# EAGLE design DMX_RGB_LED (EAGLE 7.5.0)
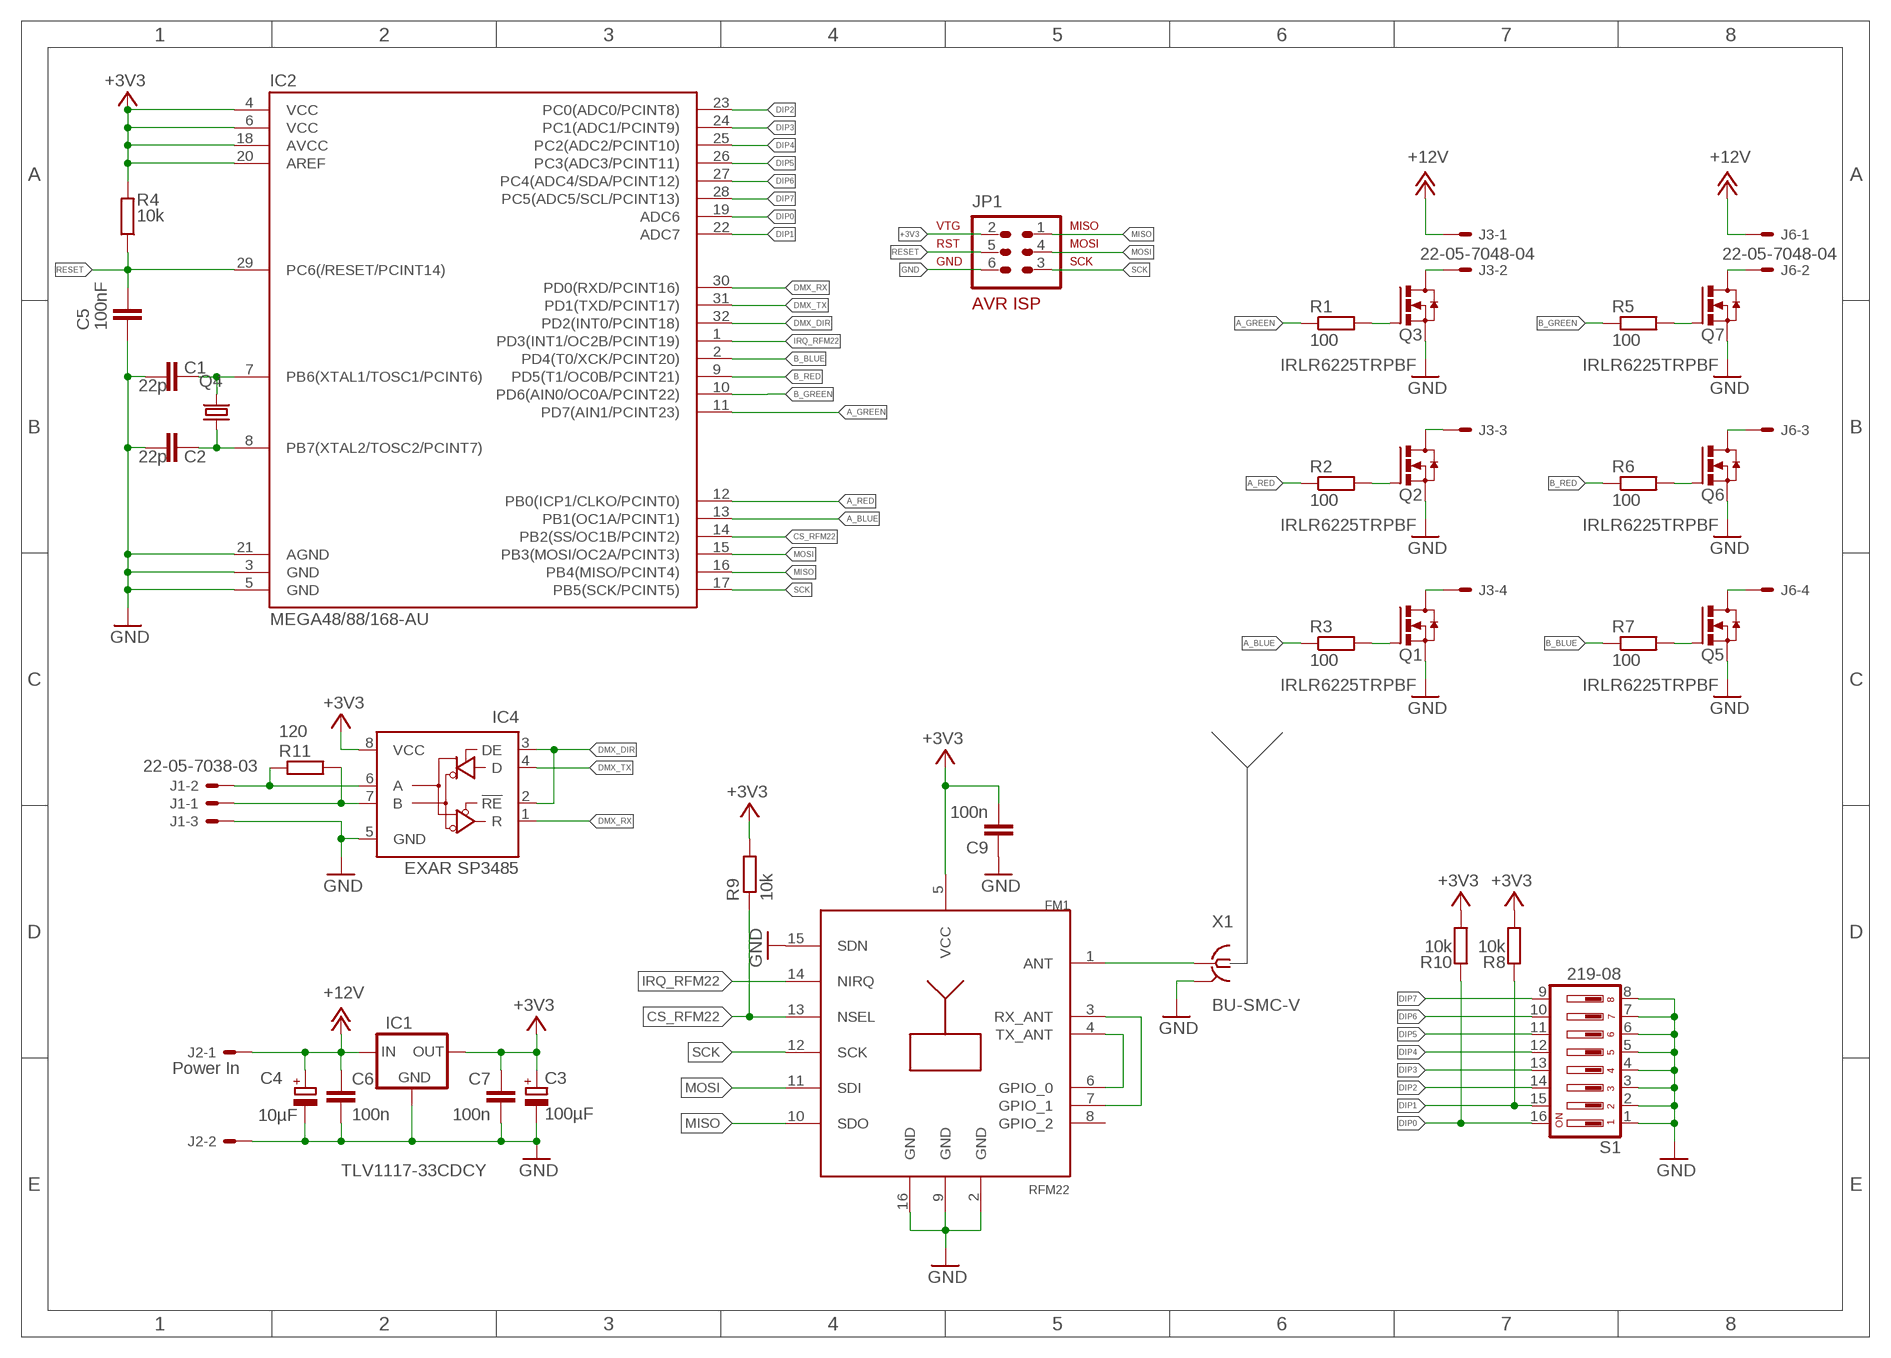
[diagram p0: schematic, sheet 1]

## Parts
C1  22p  C-EUC0805  [C0805]
C2  22p  C-EUC0805  [C0805]
C3  100µF  CPOL-EUSMCD  [SMC_D]
C4  10µF  CPOL-EUSMCD  [SMC_D]
C5  100nF  C-EUC0805  [C0805]
C6  100n  C-EUC0805  [C0805]
C7  100n  C-EUC0805  [C0805]
C9  100n  C-EUC0805  [C0805]
FM1  RFM22  [RFM22]
IC1  TLV1117-33CDCY  [DPACK]
IC2  MEGA48/88/168-AU  [TQFP32-08]
IC4  EXAR SP3485  75176AD  [D_R-PDSO-G8]
J1  22-05-7038-03  [7395-03]
J2  Power In  22-05-7028-02  [7395-02]
J3  22-05-7048-04  [7395-04]
J6  22-05-7048-04  [7395-04]
JP1  AVR-ISP-6  [AVR-ISP-6]
Q1  IRLR6225TRPBF  IRFR1205  [D-PAK_TO252AA]
Q2  IRLR6225TRPBF  IRFR1205  [D-PAK_TO252AA]
Q3  IRLR6225TRPBF  IRFR1205  [D-PAK_TO252AA]
Q4  CRYSTALCTS406  [CTS406]
Q5  IRLR6225TRPBF  IRFR1205  [D-PAK_TO252AA]
Q6  IRLR6225TRPBF  IRFR1205  [D-PAK_TO252AA]
Q7  IRLR6225TRPBF  IRFR1205  [D-PAK_TO252AA]
R1  100  R-EU_R0805  [R0805]
R2  100  R-EU_R0805  [R0805]
R3  100  R-EU_R0805  [R0805]
R4  10k  R-EU_R0805  [R0805]
R5  100  R-EU_R0805  [R0805]
R6  100  R-EU_R0805  [R0805]
R7  100  R-EU_R0805  [R0805]
R8  10k  R-EU_R0805  [R0805]
R9  10k  R-EU_R0805  [R0805]
R10  10k  R-EU_R0805  [R0805]
R11  120  R-EU_R0805  [R0805]
S1  219-08  [CTS-219-08]
X1  BU-SMC-V  [BU-SMC-V]

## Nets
+3V3: C3.+ C7.1 C9.2 FM1.5(VCC) IC1.4(OUT) IC2.4(VCC) IC2.6(VCC) IC2.18(AVCC) IC2.20(AREF) IC4.8(VCC) JP1.2 R4.2 R8.1 R9.2 R10.1
+12V: C4.+ C6.1 IC1.3(IN) J2.1 J3.1 J6.1
A_BLUE: IC2.13(PB1(OC1A/PCINT1)) R3.1
A_GREEN: IC2.11(PD7(AIN1/PCINT23)) R1.1
A_RED: IC2.12(PB0(ICP1/CLKO/PCINT0)) R2.1
B_BLUE: IC2.2(PD4(T0/XCK/PCINT20)) R7.1
B_GREEN: IC2.10(PD6(AIN0/OC0A/PCINT22)) R5.1
B_RED: IC2.9(PD5(T1/OC0B/PCINT21)) R6.1
CS_RFM22: FM1.13(NSEL) IC2.14(PB2(SS/OC1B/PCINT2)) R9.1
DIP0: IC2.19(ADC6) R10.2 S1.16
DIP1: IC2.22(ADC7) R8.2 S1.15
DIP2: IC2.23(PC0(ADC0/PCINT8)) S1.14
DIP3: IC2.24(PC1(ADC1/PCINT9)) S1.13
DIP4: IC2.25(PC2(ADC2/PCINT10)) S1.12
DIP5: IC2.26(PC3(ADC3/PCINT11)) S1.11
DIP6: IC2.27(PC4(ADC4/SDA/PCINT12)) S1.10
DIP7: IC2.28(PC5(ADC5/SCL/PCINT13)) S1.9
DMX_DIR: IC2.32(PD2(INT0/PCINT18)) IC4.2(!RE) IC4.3(DE)
DMX_RX: IC2.30(PD0(RXD/PCINT16)) IC4.1(R)
DMX_TX: IC2.31(PD1(TXD/PCINT17)) IC4.4(D)
GND: C1.1 C2.2 C3.- C4.- C5.1 C6.2 C7.2 C9.1 FM1.2(GND) FM1.9(GND) FM1.15(SDN) FM1.16(GND) IC1.1(GND) IC2.3(GND) IC2.5(GND) IC2.21(AGND) IC4.5(GND) J1.3 J2.2 JP1.6 Q1.3(S) Q2.3(S) Q3.3(S) Q5.3(S) Q6.3(S) Q7.3(S) S1.1 S1.2 S1.3 S1.4 S1.5 S1.6 S1.7 S1.8 X1.2(GND)
IRQ_RFM22: FM1.14(NIRQ) IC2.1(PD3(INT1/OC2B/PCINT19))
MISO: FM1.10(SDO) IC2.16(PB4(MISO/PCINT4)) JP1.1
MOSI: FM1.11(SDI) IC2.15(PB3(MOSI/OC2A/PCINT3)) JP1.4
N$1: Q1.1(G) R3.2
N$2: Q2.1(G) R2.2
N$3: Q3.1(G) R1.2
N$4: Q5.1(G) R7.2
N$5: Q6.1(G) R6.2
N$6: Q7.1(G) R5.2
N$8: J6.2 Q7.4(D)
N$9: J6.3 Q6.4(D)
N$10: J6.4 Q5.4(D)
N$11: FM1.1(ANT) X1.1
N$13: FM1.4(TX_ANT) FM1.6(GPIO_0)
N$14: C2.1 IC2.8(PB7(XTAL2/TOSC2/PCINT7)) Q4.1
N$15: FM1.3(RX_ANT) FM1.7(GPIO_1)
N$16: C1.2 IC2.7(PB6(XTAL1/TOSC1/PCINT6)) Q4.3
N$23: J3.2 Q3.4(D)
N$24: J3.3 Q2.4(D)
N$25: IC4.6(A) J1.2 R11.1
N$26: IC4.7(B) J1.1 R11.2
N$27: J3.4 Q1.4(D)
RESET: C5.2 IC2.29(PC6(/RESET/PCINT14)) JP1.5 R4.1
SCK: FM1.12(SCK) IC2.17(PB5(SCK/PCINT5)) JP1.3
Unconnected: FM1.8(GPIO_2)

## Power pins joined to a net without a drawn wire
GND: X1.3(GND) X1.4(GND) X1.5(GND)

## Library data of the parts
C1 C2 C5-C7 C9 = rcl:C-EU: CAPACITOR, European symbol
C3 C4 = rcl:CPOL-EU: POLARIZED CAPACITOR, European symbol
FM1 = RFMxx:RFM22
IC1 = bauteile:TLV1117-33CDCY: 500 mA Adjustable Output Positive Voltage Regulator Source: http://www.onsemi.co.jp .. LM317M-D.PDF
IC2 = bauteile:MEGA48/88/168
IC4 = 751xx:75176A: DIFFERENTIAL BUS TRANSCEIVER Source: http://focus.ti.com/lit/ds/symlink/sn75176a.pdf
J1 = con-molex:22-?-03: CONNECTOR wire to board 2.54 mm (.1 inch) pitch header; OC_FARNELL: unknown; OC_NEWARK: unknown
J2 = con-molex:22-?-02: CONNECTOR; OC_FARNELL: 9731601; OC_NEWARK: unknown
J3 J6 = con-molex:22-?-04: CONNECTOR wire to board 2.54 mm (.1 inch) pitch header; OC_FARNELL: unknown; OC_NEWARK: unknown
JP1 = avr-4:AVR-ISP-6: AVR ISP-6 Serial Programming Header
Q1-Q3 Q5-Q7 = transistor-power:IRFR1205
Q4 = crystal:CRYSTAL: CRYSTAL; OC_FARNELL: unknown; OC_NEWARK: unknown
R1-R11 = rcl:R-EU_: RESISTOR, European symbol
S1 = switch-dil:219-08*: Surface Mount DIP Switch Series 219 SMT CTS Electronic Components Sourc: www.ctscorp.com; OC_FARNELL: unknown; OC_NEWARK: unknown
X1 = con-coax:BU-SMC-V: FEMALE SMC CONNECTOR Radiall R112 426 distributor RS 295-5429

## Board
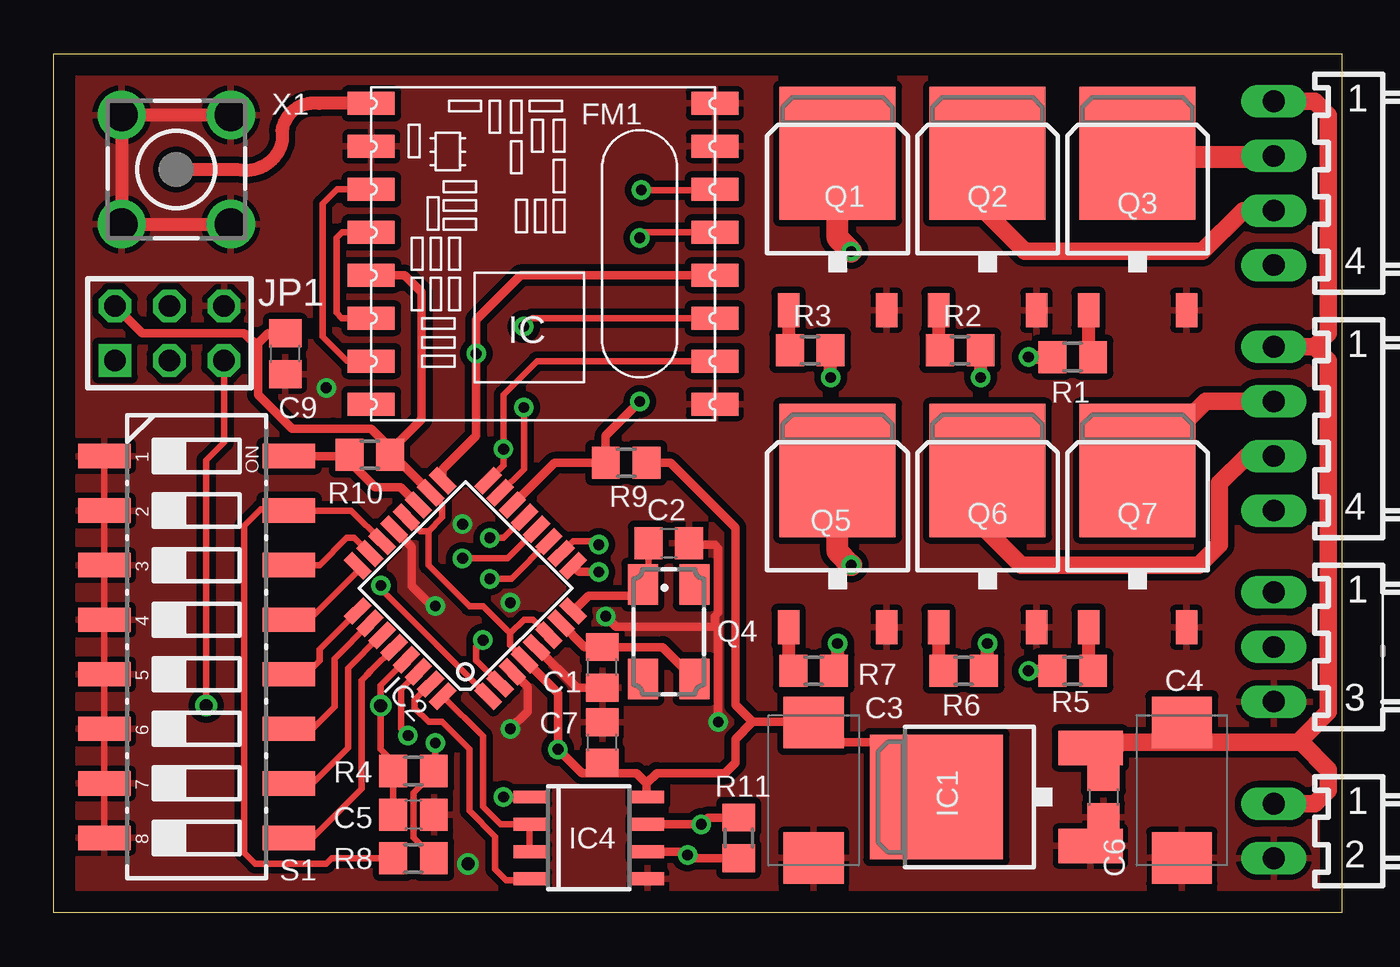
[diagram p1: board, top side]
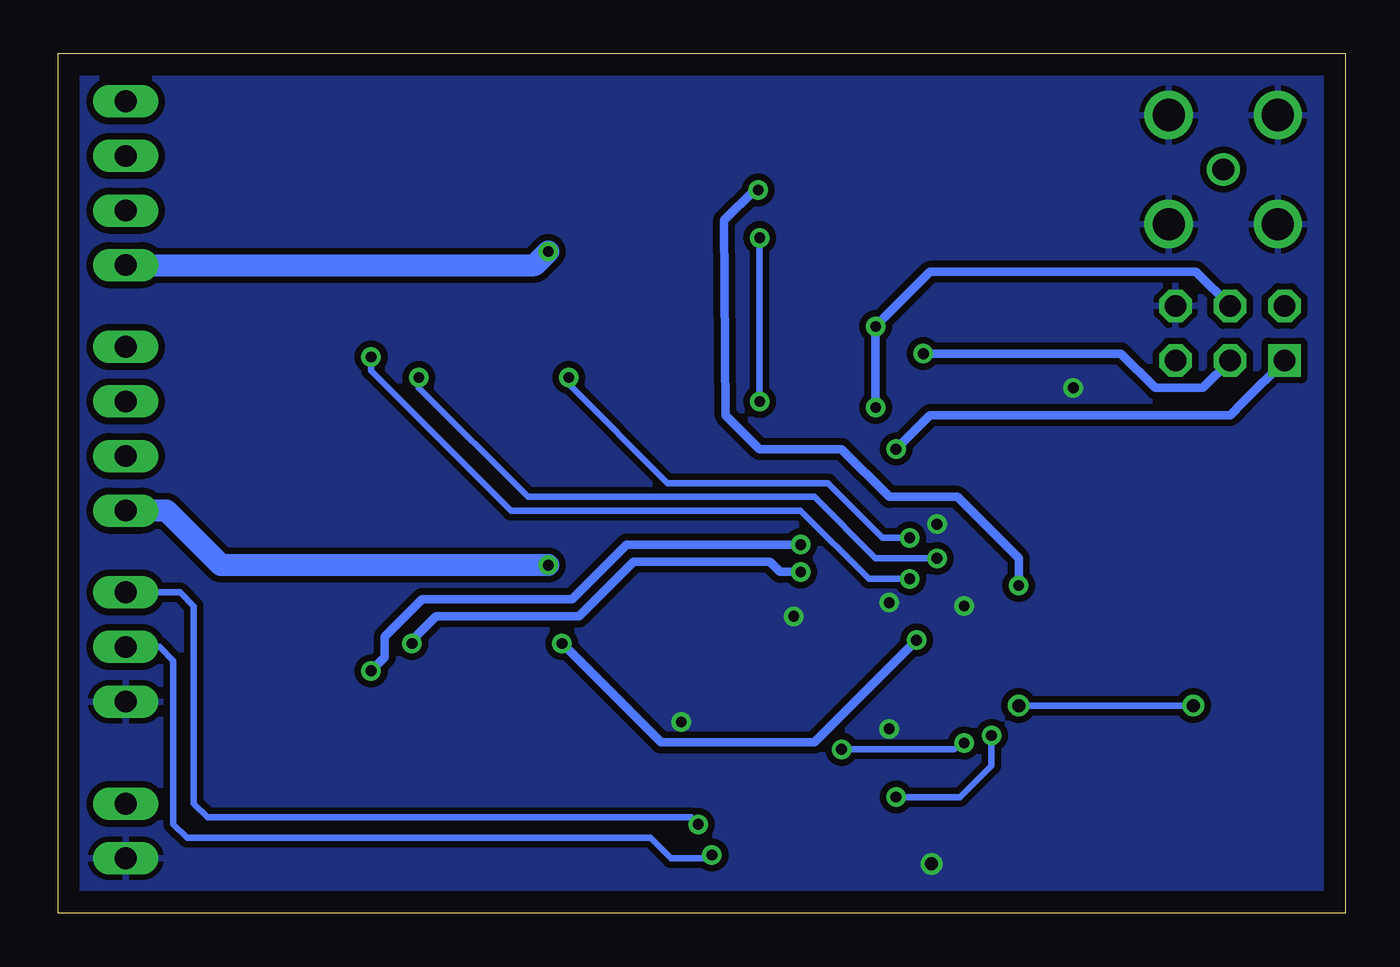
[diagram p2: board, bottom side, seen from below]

Size 60 x 40 mm. Coordinates in mm from the lower left corner, seen from the top.
Outline: 0,0 0,40 60,40 60,0 0,0
Copper layers (1*16): Top 0.035mm / dielectric 1.5mm / Bottom 0.035mm
Design rules "default": minimum track width 10mil, minimum drill 24mil, track to track 8mil, track to pad 8mil, pad to pad 8mil, via to via 8mil, smd to smd 8mil, copper to edge 40mil, drill to drill 8mil, minimum pad ring 10mil, minimum via ring 8mil, stop-mask expansion 4mil, vias tented up to drill 0mil, thermal gap 10mil

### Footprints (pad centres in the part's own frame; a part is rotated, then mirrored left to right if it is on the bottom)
C0805 = smd 1.3 x 1.5: 1 -0.95,0; 2 0.95,0
SMC_D = smd 2.4 x 2.8: + -3.15,0; - 3.15,0
RFM22 = smd 2.184 x 1.067: 1 -8.38,5.62; 2 -8.38,3.62; 3 -8.38,1.62; 4 -8.38,-0.38; 5 -8.38,-2.38; 6 -8.38,-4.38; 7 -8.38,-6.38; 8 -8.38,-8.38; 9 7.62,-8.38; 10 7.62,-6.38; 11 7.62,-4.38; 12 7.62,-2.38; 13 7.62,-0.38; 14 7.62,1.62; 15 7.625,3.625; 16 7.625,5.625
DPACK = smd 1.6 x 3: 1 -2.28,-4.8; 3 2.28,-4.8 | smd 5.8 x 6.2: 4 0,2.38
TQFP32-08 = smd 1.27 x 0.559: 1 -4.293,2.8; 2 -4.293,2; 3 -4.293,1.2; 4 -4.293,0.4; 5 -4.293,-0.4; 6 -4.293,-1.2; 7 -4.293,-2; 8 -4.293,-2.8; 17 4.293,-2.8; 18 4.293,-2; 19 4.293,-1.2; 20 4.293,-0.4; 21 4.293,0.4; 22 4.293,1.2; 23 4.293,2; 24 4.293,2.8 | smd 0.559 x 1.27: 9 -2.8,-4.293; 10 -2,-4.293; 11 -1.2,-4.293; 12 -0.4,-4.293; 13 0.4,-4.293; 14 1.2,-4.293; 15 2,-4.293; 16 2.8,-4.293; 25 2.8,4.293; 26 2,4.293; 27 1.2,4.293; 28 0.4,4.293; 29 -0.4,4.293; 30 -1.2,4.293; 31 -2,4.293; 32 -2.8,4.293
D_R-PDSO-G8 = smd 0.6 x 1.5: 1 -1.905,-2.75; 2 -0.635,-2.75; 3 0.635,-2.75; 4 1.905,-2.75; 5 1.905,2.75; 6 0.635,2.75; 7 -0.635,2.75; 8 -1.905,2.75
7395-03 = drill 1.016 long: 1 2.54,0; 2 0,0; 3 -2.54,0
7395-02 = drill 1.016 long: 1 1.27,0; 2 -1.27,0
7395-04 = drill 1.016 long: 1 3.81,0; 2 1.27,0; 3 -1.27,0; 4 -3.81,0
AVR-ISP-6 = drill 1.016 square: 1 -2.54,-1.27 | drill 1.016 octagon: 2 -2.54,1.27; 3 0,-1.27; 4 0,1.27; 5 2.54,-1.27; 6 2.54,1.27
D-PAK_TO252AA = smd 1 x 1.6: 1 -2.28,-4.8; 3 2.28,-4.8 | smd 5.4 x 6.2: 4 0,2.5
CTS406 = smd 1.9 x 1.4: 1 -2.2,-1.2; 2 2.2,-1.2; 3 2.2,1.2; 4 -2.2,1.2
R0805 = smd 1.3 x 1.5: 1 -0.95,0; 2 0.95,0
CTS-219-08 = smd 1.13 x 2.44: 1 -8.89,-4.3; 2 -6.35,-4.3; 3 -3.81,-4.3; 4 -1.27,-4.3; 5 1.27,-4.3; 6 3.81,-4.3; 7 6.35,-4.3; 8 8.89,-4.3; 9 8.89,4.3; 10 6.35,4.3; 11 3.81,4.3; 12 1.27,4.3; 13 -1.27,4.3; 14 -3.81,4.3; 15 -6.35,4.3; 16 -8.89,4.3
BU-SMC-V = drill 1.016: 1 0,0 | drill 1.5: 2 -2.54,2.54; 3 2.54,2.54; 4 2.54,-2.54; 5 -2.54,-2.54

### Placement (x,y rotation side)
C1  25.55,11.43 90 top
C2  28.64,17.21 0 top
C3  35.39,5.71 270 top
C4  52.54,5.71 270 top
C5  16.76,4.57 180 top
C6  48.89,5.39 270 top
C7  25.55,7.93 90 top
C9  10.79,26.03 90 top
FM1  23.17,32.07 0 top
IC1  43.49,5.39 90 top
IC2  19.17,15.11 135 top
IC4  24.92,3.49 270 top
J1  56.83,12.38 90 top
J2  56.83,3.81 90 top
J3  56.83,33.97 90 top
J6  56.83,22.54 90 top
JP1  5.39,26.98 0 top
Q1  36.51,32.86 0 top
Q2  43.49,32.86 0 top
Q3  50.48,32.86 0 top
Q4  28.64,13.09 270 top
Q5  36.51,18.09 0 top
Q6  43.49,18.09 0 top
Q7  50.48,18.09 0 top
R1  47.46,25.87 0 top
R2  42.22,26.19 180 top
R3  35.23,26.19 180 top
R4  16.76,6.6 0 top
R5  47.46,11.27 0 top
R6  42.38,11.27 180 top
R7  35.39,11.27 180 top
R8  16.76,2.54 180 top
R9  26.66,20.95 0 top
R10  14.72,21.33 180 top
R11  31.9,3.49 90 top
S1  6.66,12.38 270 top
X1  5.71,34.61 0 top

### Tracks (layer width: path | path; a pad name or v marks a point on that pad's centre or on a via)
+3V3  (via drill 0.5)
  Top 0.305: IC2.20 17.07,17.78 17.45,17.78 | IC2.18 18.09,19.02 18.09,18.41 17.45,17.78 | IC2.4 21.27,12.45 21.27,13.02 | IC2.6 22.33,13.65 21.9,13.65 21.27,13.02 | 17.45,17.78 17.45,16.19 19.36,14.28 20,14.28 21.27,13.02 | v17.77,7.9 17.77,6.98 R4.2 17.71,6.54 16.76,5.59 16.76,3.49 R8.1
  Top 0.406: JP1.2 4.12,26.99 8.88,26.99 9.52,26.35 | 9.52,26.35 9.52,24.13 11.11,22.54 11.42,22.54 13.01,22.54 13.96,22.54 14.57,22.54 14.79,22.54 15.49,21.84 15.49,21.52 R10.1 | FM1.5 16.34,29.69 17.14,28.89 17.14,22.98 15.99,21.84 15.99,21.65 R10.1 | 25.55,6.51 27.14,6.51 27.61,6.03 | 27.61,6.03 28.09,6.51 31.27,6.51 31.74,6.98 31.74,8.09 32.54,8.89 | 27.61,6.03 27.61,5.45 IC4.8 | 25.55,6.51 C7.1 25.55,6.51 | 32.54,8.89 35.37,8.89 C3.+ 35.39,8.73 36.19,7.94 38.57,7.94 IC1.4 | 32.54,8.89 31.74,9.68 31.74,17.94 28.73,20.95 R9.2 | 25.55,6.51 24.6,6.51 v23.49,7.62 23.49,10.23 IC2.4 | 9.52,26.35 9.52,26.51 9.99,26.99 C9.2 | IC2.18 15.78,21.33 R10.1 | 15.93,21.33 R10.1
  Bottom 0.305: v17.77,7.9 18.25,7.62 22.54,7.62 v23.49,7.62
+12V
  Top 0: 52.56,8.86 52.72,8.86
  Top 0.406: C6.1 48.89,7.08 IC1.3 48.55,7.94 | 52.51,8.86 C4.+ 52.56,8.86
  Top 0.813: J3.1 58.73,37.78 59.37,37.15 59.37,26.99 58.73,26.35 | J6.1 58.73,26.35 | 58.73,26.35 59.37,25.72 59.37,9.36 58.09,8.09 58.09,7.94 | J2.1 58.73,5.08 59.37,5.71 59.37,6.67 58.09,7.94 | 58.09,7.94 53.81,7.94 52.7,7.94 | 52.7,7.94 49.68,7.94 49.42,7.68 IC1.3 | 52.72,8.86 52.7,8.84 52.7,7.94
A_BLUE  (via drill 0.5)
  Top 0.305: v20.31,17.46 20.96,17.46 IC2.13
  Top 0.61: v36.19,24.92 R3.1
  Bottom 0.305: v20.31,17.46 21.58,17.46 24.12,20 31.58,20 36.19,24.6 v36.19,24.92
A_GREEN  (via drill 0.5)
  Top 0.305: IC2.11 21.32,15.55 20.95,15.55 v20.31,15.55
  Top 0.61: v45.4,25.87 R1.1
  Bottom 0.305: v20.31,15.55 22.22,15.55 25.39,18.73 38.89,18.73 45.4,25.24 v45.4,25.87
A_RED  (via drill 0.5)
  Top 0.305: IC2.12 21.14,16.51 20.95,16.51 v19.04,16.51
  Top 0.61: v43.17,24.92 R2.1
  Bottom 0.305: v19.04,16.51 21.9,16.51 24.76,19.36 38.09,19.36 43.17,24.45 v43.17,24.92
B_BLUE  (via drill 0.5)
  Top 0.305: IC2.2 19.71,11.75 19.68,11.75 19.68,12.38 v20,12.7
  Top 0.406: 36.5,11.27 R7.1
  Top 0.61: v36.51,12.54 36.5,11.27
  Bottom 0.406: v36.51,12.54 36.19,12.22 31.9,7.94 27.61,7.94 24.76,7.94 v20,12.7
B_GREEN  (via drill 0.5)
  Top 0.305: IC2.10 24.2,17.3 25.23,17.3 | v25.39,17.14 25.23,17.3 | 25.23,17.3 v25.39,17.14 | v25.39,17.14 25.23,17.3
  Top 0.61: v45.4,11.27 R5.1
  Bottom 0.406: v25.39,17.14 26.34,17.14 33.49,17.14 36.03,14.6 43.01,14.6 44.76,12.86 44.76,11.9 v45.4,11.27
B_RED  (via drill 0.5)
  Top 0.406: v25.39,15.87 24.48,15.87 IC2.9 | R6.1 43.49,11.27 | v43.49,12.54
  Top 0.61: 43.49,11.27 v43.49,12.54
  Bottom 0.406: v25.39,15.87 26.34,15.87 26.82,16.35 33.17,16.35 35.71,13.81 42.38,13.81 42.54,13.65 43.49,12.7 v43.49,12.54
CS_RFM22  (via drill 0.5)
  Top 0.305: FM1.13 27.55,31.69 v27.3,31.43
  Top 0.406: IC2.14 23.32,20.95 R9.1 25.71,22.22 v27.3,23.81
  Bottom 0.305: v27.3,31.43 v27.3,23.81
DIP0
  Top 0.406: S1.16 13.77,21.27 R10.2 13.77,21.01 14.98,19.81 15.23,19.81 16.17,19.81 IC2.19
DIP1
  Top 0.305: IC2.22 13.85,18.73 S1.15 10.9,18.79 9.64,18.79 8.88,18.03 8.88,2.79 9.39,2.28 12.69,2.28 12.95,2.54 R8.2
DIP2
  Top 0.305: IC2.23 13.99,17.46 13.64,17.46 12.38,16.19 S1.14
DIP3
  Top 0.305: 14.16,15.91 11.9,13.65 S1.13
  Top 0.406: IC2.24 14.16,15.91
DIP4
  Top 0.305: IC2.25 12.38,12.27 12.38,11.75 11.74,11.11 S1.12
DIP5
  Top 0.305: S1.11 12.06,8.57 13.07,9.59 13.07,10.95 13.07,11.83 IC2.26
DIP6
  Top 0.305: IC2.27 15.23,12.92 13.71,11.4 13.71,7.68 12.06,6.03 S1.10
DIP7
  Top 0.305: IC2.28 14.76,11.26 | 14.76,11.26 14.6,11.1 | S1.9 12.06,3.49 14.34,5.78 14.34,10.84 14.76,11.26
DMX_DIR
  Top 0.305: IC2.32 20,8.21 20,4.95 20.82,4.13 IC4.2 IC4.3
DMX_RX  (via drill 0.5)
  Top 0.305: IC2.30 16.18,10.42 16.18,8.57 v16.5,8.25
  Top 0.406: v20.95,5.39 IC4.1
  Bottom 0.305: v20.95,5.39 17.96,5.39 16.5,6.86 v16.5,8.25
DMX_TX
  Top 0.305: IC2.31 16.82,9.92 16.82,9.52 17.45,8.89 18.09,8.89 19.36,7.62 19.36,4.76 20.57,3.55 20.57,2.03 21.07,1.52 22.1,1.52 IC4.4
GND  (via drill 0.5, 0.6)
  Top 0.305: S1.8 S1.7 S1.6 S1.5 S1.4 S1.3 S1.2 S1.1
  Top 0.406: IC2.21 16.66,17.05 16.66,15.24 17.61,14.28 v17.77,14.28 | IC2.3 22.06,10.52 22.06,9.36 v21.27,8.57 | IC2.5 24.37,10.48 C1.1 | v25.71,13.81 26.19,13.33 30.95,13.33 v30.95,8.89 | 30.79,13.33 30.79,13.81 30.95,13.97 30.95,16.98 30.79,17.14 29.67,17.14 C2.2
  Top 0.61: X1.4 X1.5 X1.2 X1.3
  other vias: 19.04,18.09 21.27,14.44 12.69,24.45 19.3,2.28
  pour Top (isolate 0.305): 0,40 60,40 60,0 0,0
  pour Bottom (isolate 0.305): 0,40 60,40 60,0 0,0
IRQ_RFM22  (via drill 0.5)
  Top 0.305: IC2.1 15.23,15.09 v15.23,15.24 | v27.36,33.65 30.76,33.65 FM1.14
  Bottom 0.406: v15.23,15.24 15.23,16.51 18.09,19.36 21.27,19.36 23.49,21.59 27.3,21.59 28.88,23.17 28.95,32.26 27.55,33.65 v27.36,33.65
MISO  (via drill 0.5)
  Top 0.305: IC2.16 20.95,20.84 20.95,21.27 v20.95,21.59 20.95,24.13 22.5,25.69 FM1.10
  Bottom 0.406: JP1.1 4.76,23.81 5.39,23.17 19.36,23.17 v20.95,21.59
MOSI  (via drill 0.5)
  Top 0.305: IC2.15 21.9,20.66 v21.9,23.52 | v21.9,27.3 22.28,27.69 FM1.11
  Bottom 0.406: JP1.4 6.98,29.84 19.36,29.84 v21.9,27.3 v21.9,23.52
N$1
  Top 0.406: 34.23,25.93 R3.2
  Top 0.61: Q1.1 34.23,25.93
N$2
  Top 0.61: Q2.1 41.21,25.93 R2.2
N$3
  Top 0.406: 48.2,25.93 48.25,25.87 R1.2
  Top 0.61: Q3.1 48.2,25.93
N$4
  Top 0.406: 34.23,11.27 R7.2
  Top 0.61: Q5.1 34.23,11.27
N$5
  Top 0.406: 41.21,11.27 R6.2
  Top 0.61: Q6.1 41.21,11.27
N$6
  Top 0.406: 48.2,11.11 R5.2
  Top 0.61: Q7.1 48.2,11.11
N$8
  Top 0.813: Q7.4 50.48,20.63 53.65,23.81 J6.2 57.46,23.81
N$9
  Top 0.813: Q6.4 43.49,17.78 45.08,16.19 53.33,16.19 54.28,17.14 54.28,20 55.55,21.27 J6.3 | J6.3 57.46,21.27 J6.3
N$10  (via drill 0.5)
  Top 1.016: Q5.4 36.51,16.83 v37.14,16.19
  Bottom 1.016: v37.14,16.19 52.38,16.19 54.92,18.73 J6.4
N$11
  Top 0.61: X1.1 8.56,34.61 arc90 10.63,35.87 10.63,36.41 arc-90 12.38,37.69 FM1.1
N$13
  Top 0.305: FM1.6 13.42,27.69 13.17,27.94 13.17,31.43 13.42,31.69 FM1.4
N$14
  Top 0.305: Q4.1 27.7,15.54 C2.1
  Top 0.406: IC2.8 24.9,14.76 27.46,14.76 27.45,14.77 Q4.1
N$15
  Top 0.305: FM1.3 13.2,33.69 12.53,33.02 12.53,26.83 13.64,25.72 14.76,25.72 FM1.7
N$16
  Top 0.406: IC2.7 24.73,12.38 C1.2 28.36,12.38 Q4.3
N$23
  Top 0.813: 56.78,35.2 J3.2
  Top 1.016: Q3.4 50.48,35.24 50.52,35.2 56.78,35.2
N$24
  Top 0.813: Q2.4 43.49,32.54 45.24,30.79 53.49,30.79 55.4,32.7 J3.3
N$25  (via drill 0.5)
  Top 0.406: IC4.6 29.36,2.85 v29.52,2.7 29.68,2.54 30.15,2.54 R11.1
  Bottom 0.305: J1.2 55.24,12.38 54.6,11.75 54.6,4.13 53.97,3.49 32.38,3.49 31.43,2.54 29.68,2.54 v29.52,2.7
N$26  (via drill 0.5)
  Top 0.305: 32.06,4.44 R11.2
  Top 0.406: IC4.7 28.41,4.13 v30.16,4.13 30.47,4.44 R11.2
  Bottom 0.305: v30.16,4.13 30.47,4.44 53.02,4.44 53.65,5.08 53.65,14.28 54.28,14.92 J1.1
N$27  (via drill 0.5)
  Top 1.016: Q1.4 36.51,31.43 v37.14,30.79
  Bottom 1.016: J3.4 37.77,30.16 v37.14,30.79
RESET  (via drill 0.6)
  Top 0.305: IC2.29 15.55,10.92 15.23,10.6 v15.23,9.65 15.23,7.62 15.49,7.36 15.74,7.11 15.74,6.16 R4.1 | R4.1 15.55,6.03 | R4.1 C5.2 15.87,4.5 | JP1.5 7.93,21.9 7.1,21.08 v7.1,9.65 | v7.1,9.65 7.17,9.71 v7.1,9.65
  Bottom 0.305: v7.1,9.65 v15.23,9.65 15.3,9.65
SCK  (via drill 0.5)
  Top 0.406: IC2.17 18.12,20.66 19.68,22.22 v19.68,26.03 19.68,27.62 21.74,29.69 FM1.12
  Bottom 0.406: JP1.3 6.66,24.45 8.88,24.45 10.47,26.03 v19.68,26.03

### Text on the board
text: +12V | CH6 BLAU | CH5 GRÜN | CH4 ROT | +12V | CH3 BLAU | CH2 GRÜN | CH1 ROT | DMX- | DMX+ | GND | + | max. 12Volt | -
